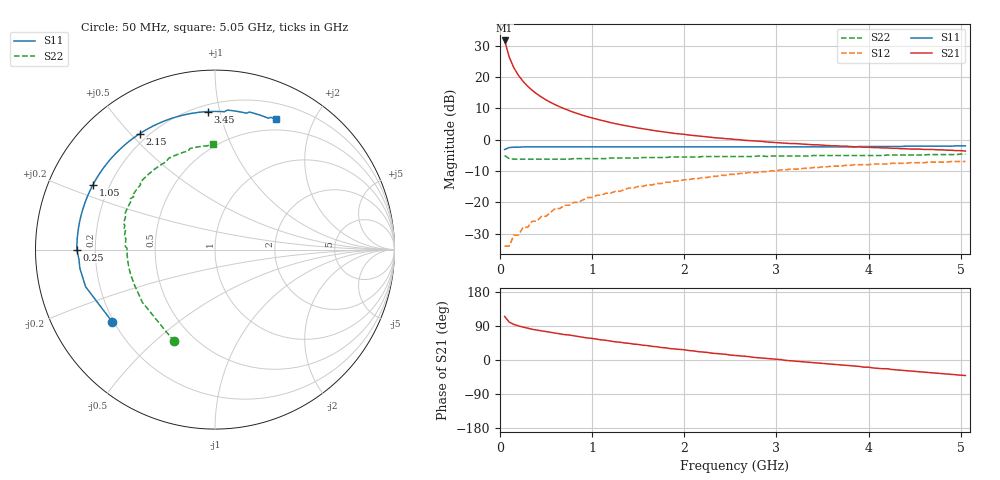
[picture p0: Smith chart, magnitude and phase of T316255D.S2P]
!AT-31625
!S-PARAMETERS at Vce=4.8 V  Ic=200 mA.  LAST UPDATED 08-05-96
# ghz s ma r 50
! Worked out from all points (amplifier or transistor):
!   101 points, 50 MHz to 5.05 GHz, reference 50 ohm
!   highest |S21| = 31.7 dB at 50 MHz (marker M1)
!   |S21| within 3 dB of that: start of sweep to 78.3 MHz
!   unconditionally stable (mu >= 1): 397.9 MHz to 407.5 MHz; 463.7 MHz to 595.2 MHz; 601.6 MHz to 1.792 GHz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
!   at 850 MHz: K = 1.05, MAG = 12.7 dB, |S12| = -20.0 dB
!   at 2.55 GHz: K = 0.97, MSG = 5.6 dB, |S12| = -11.1 dB
!   at 5.05 GHz: K = 0.95, MSG = 1.7 dB, |S12| = -6.9 dB
!   S11 on the Smith chart (normalised r, x): 50 MHz: 0.19, -0.30; 250 MHz: 0.13, -0.00; 1.05 GHz: 0.14, +0.24; 2.15 GHz: 0.17, +0.53; 3.45 GHz: 0.24, +0.92; 5.05 GHz: 0.37, +1.50
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0.05  0.7 -145.0  38.47 115.0  0.02 41.0  0.56 -114.0
0.1  0.75 -164.0  20.9 100.0  0.02 43.0  0.5 -144.0
0.15  0.76 -172.0  14.14 94.0  0.03 49.0  0.49 -156.0
0.2  0.76 -176.0  10.67 90.0  0.03 53.0  0.49 -163.0
0.25  0.77 -180.0  8.57 87.0  0.04 57.0  0.49 -167.0
0.3  0.77 178.0  7.16 84.0  0.04 59.0  0.49 -170.0
0.35  0.77 175.0  6.15 81.0  0.05 61.0  0.49 -172.0
0.4  0.77 173.0  5.38 79.0  0.05 62.0  0.49 -173.0
0.45  0.77 171.0  4.8 77.0  0.06 63.0  0.49 -175.0
0.55  0.77 168.0  3.94 73.0  0.07 64.0  0.49 -177.0
0.65  0.77 164.0  3.35 69.0  0.08 64.0  0.49 -180.0
0.8  0.77 160.0  2.74 64.0  0.1 63.0  0.5 178.0
0.9  0.77 157.0  2.45 60.0  0.11 62.0  0.5 176.0
1.05  0.77 152.0  2.13 55.0  0.13 61.0  0.5 174.0
1.35  0.77 144.0  1.69 45.0  0.16 56.0  0.51 170.0
1.75  0.77 134.0  1.35 33.0  0.2 50.0  0.52 165.0
2.15  0.77 123.0  1.15 22.0  0.24 43.0  0.53 160.0
2.55  0.77 114.0  1.01 12.0  0.28 36.0  0.54 154.0
3.4  0.77 94.0  0.83 -7.0  0.36 20.0  0.56 138.0
3.45  0.77 93.0  0.83 -8.0  0.36 19.0  0.56 137.0
4.25  0.78 79.0  0.73 -25.0  0.42 2.0  0.57 116.0
5.05  0.8 65.0  0.66 -41.0  0.45 -14.0  0.59 91.0
